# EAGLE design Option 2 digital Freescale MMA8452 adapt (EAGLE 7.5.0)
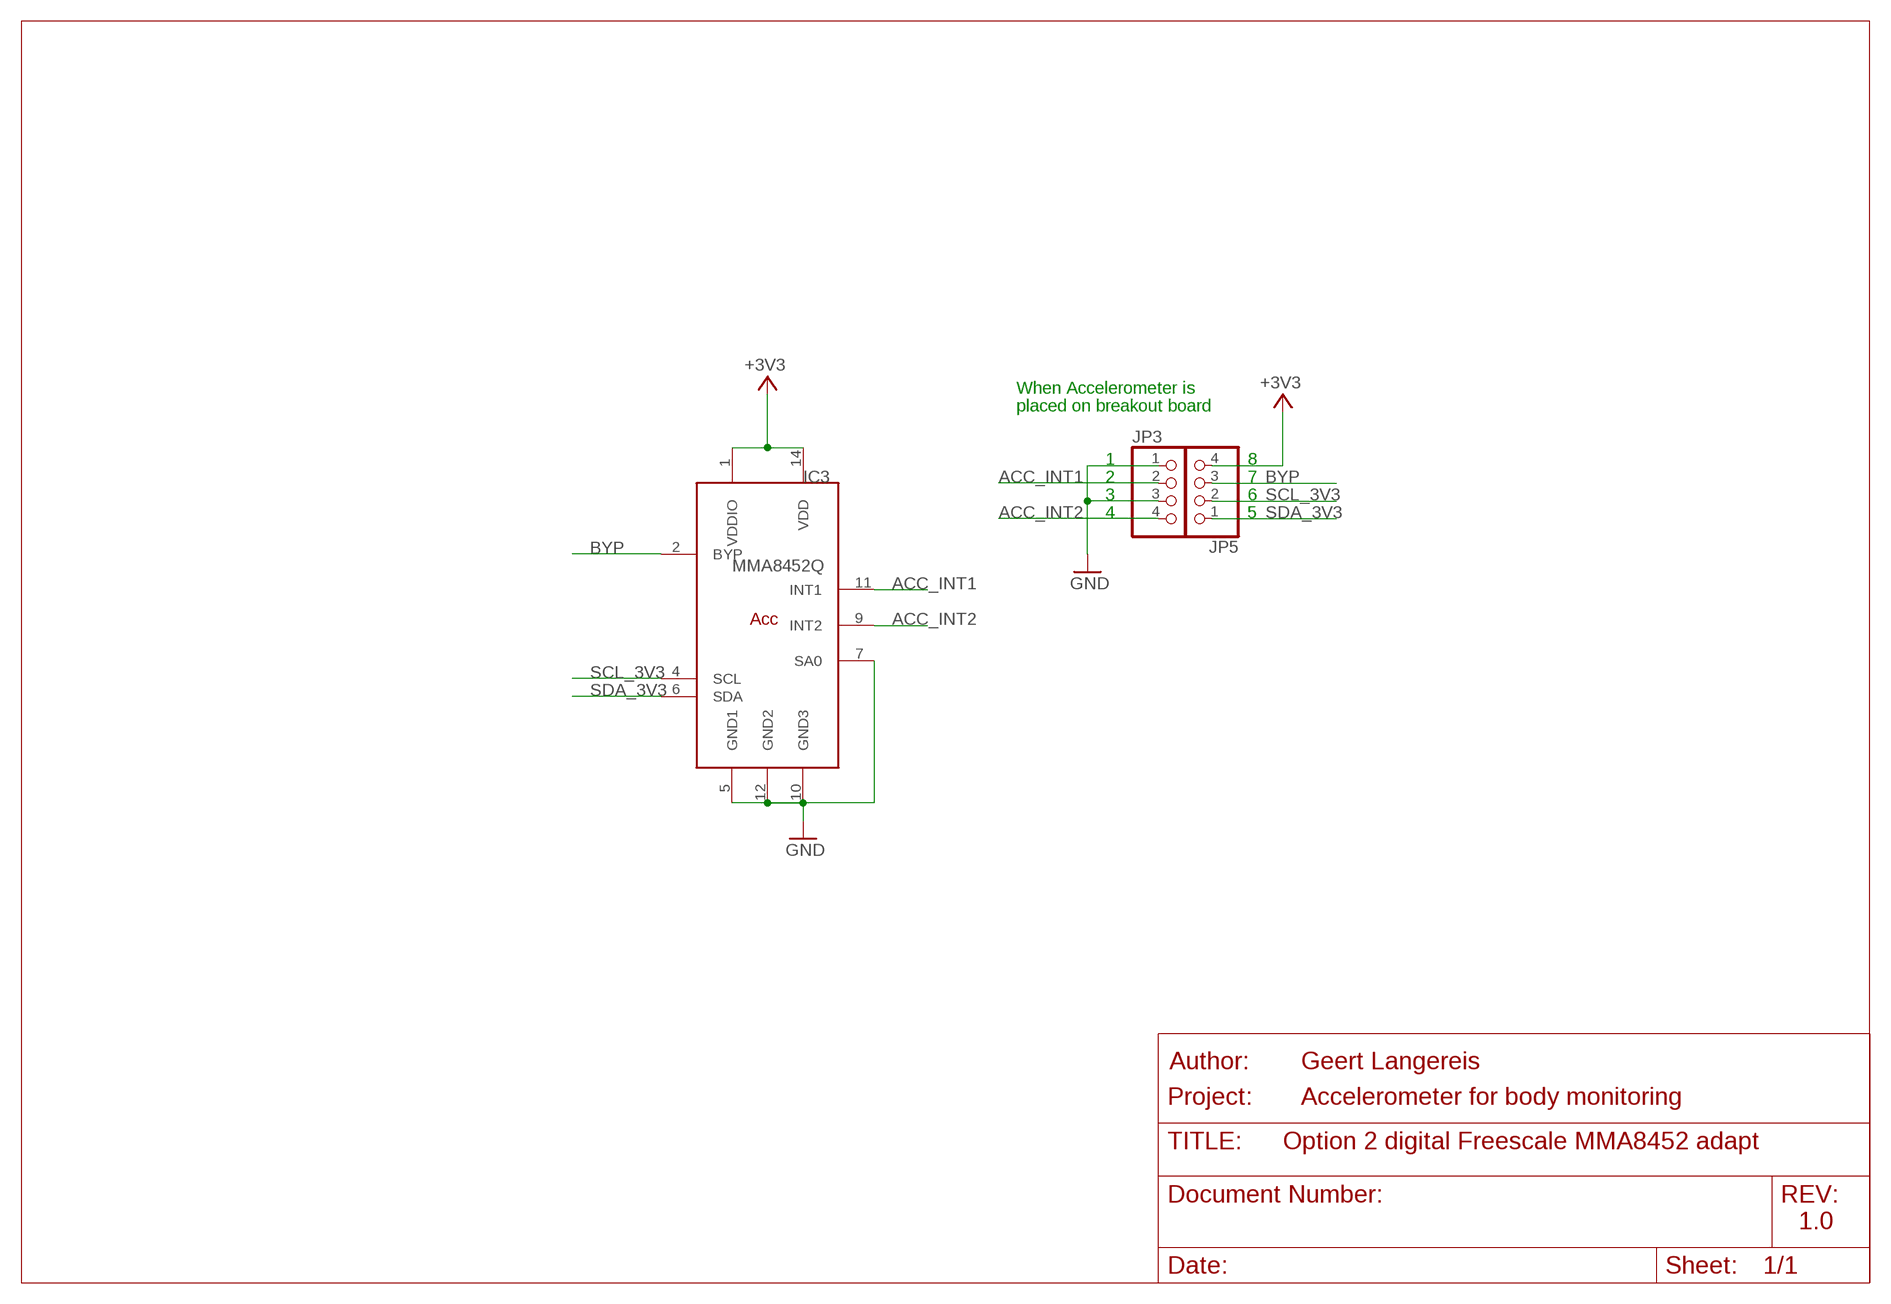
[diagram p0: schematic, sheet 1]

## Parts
IC3  MMA8452Q  [QFN-16]
JP3  PINHD-1X4  [1X04]
JP5  PINHD-1X4  [1X04]

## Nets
+3V3 [usbvcc]: IC3.1(VDDIO) IC3.14(VDD) JP5.4
ACC_INT1: IC3.11(INT1) JP3.2
ACC_INT2: IC3.9(INT2) JP3.4
BYP: IC3.2(BYP) JP5.3
GND [gnd]: IC3.5(GND1) IC3.7(SA0) IC3.10(GND3) IC3.12(GND2) JP3.1 JP3.3
SCL_3V3: IC3.4(SCL) JP5.2
SDA_3V3: IC3.6(SDA) JP5.1

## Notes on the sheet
- When Accelerometer is
- placed on breakout board
- 1 | 8
- 2 | 7
- 3 | 6
- 4 | 5
- Geert Langereis
- Accelerometer for body monitoring
- 1.0

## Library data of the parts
IC3 = Geert-library:MMA8452Q: 3-Axis, 12-bit/8-bit Digital Accelerometer (Freescale)
JP3 JP5 = pinhead:PINHD-1X4: PIN HEADER

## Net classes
0 default: width 0.254 mm, drill 0.305 mm, clearance 0.152 mm
1 power: width 0.61 mm, drill 0.508 mm, clearance 0.152 mm
2 gnd: width 0.305 mm, drill 0.508 mm, clearance 0.152 mm
3 usbvcc: width 0.508 mm, drill 0.508 mm, clearance 0.152 mm
4 aref: width 0.406 mm

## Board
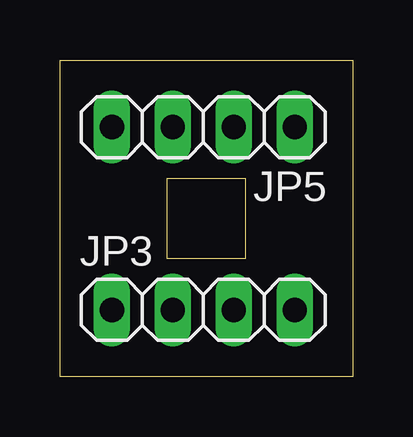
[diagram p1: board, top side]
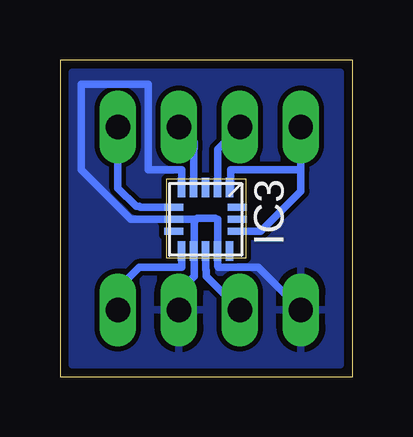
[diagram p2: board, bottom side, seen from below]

Size 12.19 x 13.21 mm. Coordinates in mm from the lower left corner, seen from the top.
Outline: 0,0 0,13.21 12.19,13.21 12.19,0 0,0
Copper layers (1*16): Top 0.035mm / dielectric 1.5mm / Bottom 0.035mm
Design rules "default *": minimum track width 10mil, minimum drill 24mil, track to track 8mil, track to pad 8mil, pad to pad 8mil, via to via 8mil, smd to smd 8mil, copper to edge 8mil, drill to drill 8mil, minimum pad ring 10mil, minimum via ring 8mil, stop-mask expansion 4mil, vias tented up to drill 0mil, thermal gap 10mil

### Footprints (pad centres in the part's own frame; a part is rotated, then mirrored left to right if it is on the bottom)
QFN-16 = smd 0.8 x 0.3: 1 -3.325,3; 2 -3.325,2.5; 3 -3.325,2; 4 -3.325,1.5; 5 -3.325,1; 9 -0.675,1; 10 -0.675,1.5; 11 -0.675,2; 12 -0.675,2.5; 13 -0.675,3 | smd 0.3 x 0.8: 6 -2.5,0.675; 7 -2,0.675; 8 -1.5,0.675; 14 -1.5,3.325; 15 -2,3.325; 16 -2.5,3.325
1X04 = drill 1.016 long: 1 -3.81,0; 2 -1.27,0; 3 1.27,0; 4 3.81,0

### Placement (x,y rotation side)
IC3  8.13,4.57 270 bottom
JP3  5.97,2.79 0 top
JP5  5.97,10.41 180 top

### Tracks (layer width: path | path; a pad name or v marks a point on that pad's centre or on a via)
+3V3
  Bottom 0.305: 2.16,8.64 JP5.4 | IC3.1 5.08,7.9 5.08,8.64 2.16,8.64 | IC3.14 3.83,6.07 2.16,7.75 2.16,8.64
ACC_INT1
  Bottom 0.305: IC3.11 6.13,4.48 6.1,4.45 6.1,4.19 JP3.2
ACC_INT2
  Bottom 0.305: IC3.9 7.13,4.59 7.11,4.57 8.89,4.57 9.78,3.68 JP3.4
BYP
  Bottom 0.305: IC3.2 5.63,9.48 JP5.3
GND
  Bottom 0.305: JP3.1 3.94,4.57 5.59,4.57 5.63,4.61 IC3.12 5.63,6.56 5.72,6.6 6.48,6.6 6.6,6.48 | JP3.3 7.24,3.56 6.6,4.19 6.6,5.22 IC3.10 6.6,5.27 6.6,6.48 | 6.6,6.48 6.57,6.57 IC3.7 9.24,6.57 11.3,8.64 11.3,12.19 8.51,12.19 8.51,8.64 7.11,8.64 7.11,7.91 IC3.5
  pour Bottom: 0.51,12.7 11.68,12.7 11.68,0.51 0.51,0.51
SCL_3V3
  Bottom 0.305: IC3.4 6.63,9.5 6.6,9.52 6.6,9.78 JP5.2
SDA_3V3
  Bottom 0.305: IC3.6 8.85,7.07 8.89,7.11 9.02,7.11 9.78,7.87 JP5.1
